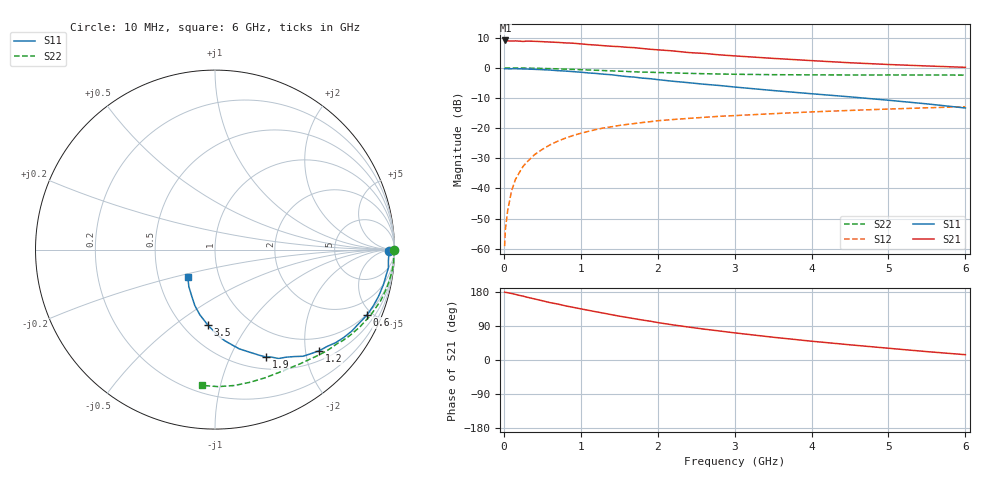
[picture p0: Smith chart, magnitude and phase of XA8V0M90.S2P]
! SIEMENS Discrete & RF Semiconductors
! BFY180
! Si NPN RF Bipolar Junction Transistor in MICRO-X
! VCE = 8 V  IC = 0.9 mA
! Common Emitter S-Parameters:  May  1997
# GHz  S  MA  R  50
!  f  S11  S21  S12  S22
! GHz  MAG  ANG  MAG  ANG  MAG  ANG  MAG  ANG
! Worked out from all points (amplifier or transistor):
!   36 points, 10 MHz to 6 GHz, reference 50 ohm
!   highest |S21| = 9.1 dB at 20 MHz (marker M1)
!   |S21| within 3 dB of that: start of sweep to 1.945 GHz
!   unconditionally stable (mu >= 1): 4.5 GHz to end of sweep
!   at 250 MHz: K = 0.08, MSG = 20.7 dB, |S12| = -32.7 dB
!   at 1.4 GHz: K = 0.46, MSG = 13.4 dB, |S12| = -19.5 dB
!   at 6 GHz: K = 1.04, MAG = 5.4 dB, |S12| = -12.9 dB
!   S11 on the Smith chart (normalised r, x): 10 MHz: 60, -13; 600 MHz: 0.96, -4.66; 1.2 GHz: 0.70, -2.29; 1.9 GHz: 0.65, -1.38; 3.5 GHz: 0.65, -0.67; 6 GHz: 0.71, -0.23
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0.01  0.9685 -0.4  2.804 179.1  0.0011 77.0  0.9984 -0.1
0.02  0.9702 -0.7  2.857 178.4  0.0021 97.4  0.999 -0.5
0.05  0.9687 -1.8  2.81 177.6  0.0043 86.7  0.998 -1.2
0.1  0.9682 -3.9  2.791 175.5  0.0091 89.2  0.9961 -2.5
0.15  0.9717 -6.0  2.808 173.2  0.014 86.7  0.9972 -3.8
0.25  0.9616 -9.8  2.752 168.5  0.0232 82.7  0.995 -6.4
0.3  0.9582 -11.9  2.786 165.8  0.0274 81.3  0.9916 -7.6
0.6  0.9219 -23.3  2.688 151.4  0.0528 73.2  0.9727 -14.9
0.9  0.8681 -34.4  2.571 139.0  0.0756 65.1  0.9451 -21.8
1.1  0.8255 -40.8  2.441 131.1  0.0886 60.5  0.9242 -26.0
1.2  0.8096 -44.1  2.396 127.2  0.095 58.1  0.9148 -28.1
1.5  0.7423 -53.4  2.256 115.7  0.111 52.1  0.8833 -33.8
1.7  0.7032 -59.7  2.168 108.9  0.1195 48.6  0.861 -37.2
1.9  0.663 -64.5  2.042 102.5  0.128 45.4  0.8468 -40.5
2.2  0.6006 -71.7  1.915 92.6  0.1392 41.1  0.8256 -45.2
2.6  0.5365 -80.2  1.742 81.5  0.1512 36.4  0.8016 -50.7
3  0.4819 -87.7  1.583 71.6  0.1616 32.2  0.7849 -55.9
3.5  0.4217 -95.5  1.441 60.1  0.1741 27.8  0.7722 -62.2
4  0.3728 -103.1  1.322 49.6  0.1861 23.4  0.7667 -68.6
4.5  0.331 -109.9  1.218 40.1  0.1971 19.3  0.7645 -75.1
5.5  0.2531 -125.1  1.078 22.1  0.2178 11.2  0.7636 -88.7
6  0.2161 -134.5  1.023 14.0  0.2271 6.9  0.76 -95.6
